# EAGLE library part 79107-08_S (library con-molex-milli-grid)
RECEPTACAL
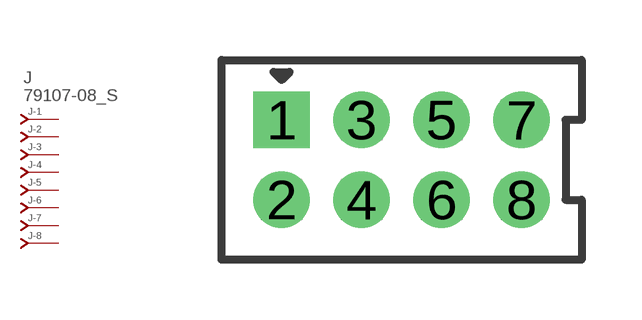
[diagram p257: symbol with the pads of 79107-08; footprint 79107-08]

Designator prefix J; gates -1=J-NV -2=J-N -3=J-N -4=J-N -5=J-N -6=J-N -7=J-N -8=J-N

## 79107-08_S  [79107-08]
1  -1:J  pas
2  -2:J  pas
3  -3:J  pas
4  -4:J  pas
5  -5:J  pas
6  -6:J  pas
7  -7:J  pas
8  -8:J  pas

## Footprint 79107-08 (pad centres in mm)
RECEPTACAL Dual Row, Vertical, Through-Hole
drill 0.914 square: 1 -3,1
drill 0.914: 2 -3,-1; 3 -1,1; 4 -1,-1; 5 1,1; 6 1,-1; 7 3,1; 8 3,-1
